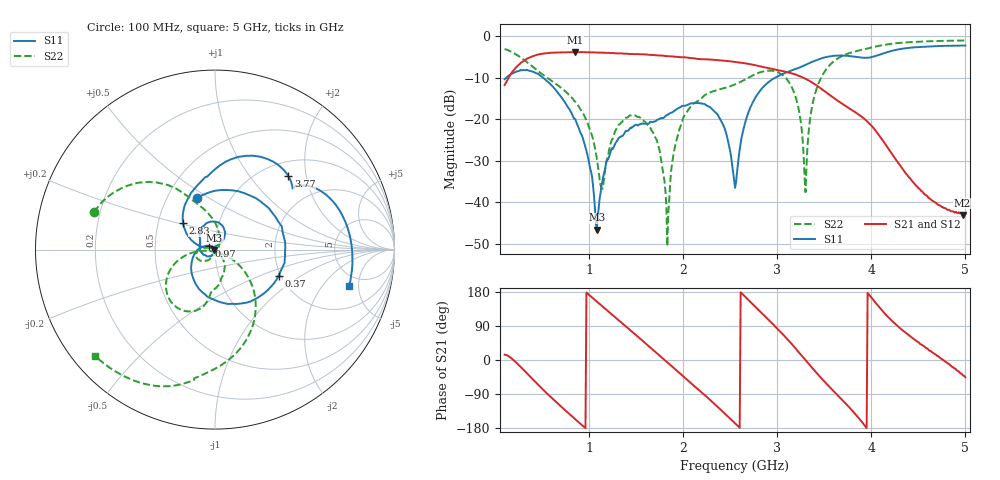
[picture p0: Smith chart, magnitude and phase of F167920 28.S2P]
!  2-Port S-parameters saved by WinCal
! VAR MeasName=S-Parameters (CALIBRATED_DATA) read from VNA (N5242A)
! VAR MeasDate=2016-11-22 9:56:32
! VAR NAME=F167920 28
! VAR FILENAME=F167920 28.S2P
! VAR DATE=2016-11-22 9:56:32
! VAR PHYS_PORTS=1,2
# Hz S DB R 50
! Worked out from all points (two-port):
!   491 points, 100 MHz to 5 GHz, reference 50 ohm
!   highest |S21| = -3.78 dB at 850 MHz (marker M1); lowest = -43.1 dB at 4.97 GHz (marker M2)
!   |S21| within 3 dB of the highest: 254.8 MHz to 2.725 GHz (2.47 GHz wide, 166 % of centre)
!   lowest |S11| = -46.7 dB at 1.08 GHz (marker M3), VSWR 1.01, Z = 49.6 - j0.172 ohm
!   |S11| at or under -10 dB: start of sweep to 116.4 MHz; 509.2 MHz to 2.976 GHz (2.466 GHz wide, 142 % of centre)
!   |S22| runs from -50.6 to -1.0 dB; largest |S21 - S12| = 0.0011
!   S11 on the Smith chart (normalised r, x): 100 MHz: 0.70, +0.45; 370 MHz: 1.95, -0.66; 970 MHz: 0.93, +0.04; 2.83 GHz: 0.67, +0.21; 3.77 GHz: 1.28, +1.58; 5 GHz: 3.77, -3.87
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1e8  -10.32 109.2  -11.75 14.3  -11.75 14.3  -3.05 162.8
3.7e8  -8.34 -22.4  -5.06 -43.5  -5.06 -43.4  -6.79 127.5
5.9e8  -11.57 -99.8  -3.96 -97.8  -3.95 -97.8  -10.61 113.7
8.5e8  -19.93 -177.9  -3.78 -156.1  -3.78 -156.1  -15.73 93.5
9.2e8  -23.80 164.6  -3.79 -171.1  -3.79 -171.1  -18.15 84.9
9.7e8  -27.62 149.8  -3.83 178.0  -3.83 178.0  -20.25 77.1
1.08e9  -46.65 -158.1  -3.90 154.4  -3.90 154.4  -29.36 45.7
1.14e9  -35.01 -107.6  -3.93 141.5  -3.93 141.5  -36.80 -39.0
1.3e9  -25.05 -137.6  -4.11 107.5  -4.11 107.5  -21.83 -129.5
1.74e9  -20.03 146.6  -4.60 13.4  -4.60 13.4  -26.86 165.8
1.83e9  -18.87 138.9  -4.77 -5.9  -4.76 -5.9  -50.63 -132.6
2.02e9  -16.75 115.5  -5.06 -47.4  -5.07 -47.4  -18.86 -62.1
2.37e9  -19.08 59.4  -5.74 -124.6  -5.75 -124.7  -12.87 -92.8
2.55e9  -36.55 102.8  -6.14 -166.9  -6.15 -166.9  -11.61 -96.9
2.83e9  -12.73 140.4  -7.28 124.8  -7.29 124.8  -8.58 -112.2
3.16e9  -8.16 100.8  -8.97 40.5  -8.98 40.5  -12.55 -161.0
3.3e9  -6.88 89.2  -10.23 -0.4  -10.24 -0.4  -37.60 -83.7
3.37e9  -6.14 83.2  -11.12 -20.6  -11.14 -20.6  -16.87 -31.8
3.77e9  -4.75 45.1  -17.44 -126.2  -17.47 -126.1  -4.01 -84.7
4.19e9  -3.66 31.4  -27.40 110.5  -27.44 110.8  -1.86 -109.3
4.97e9  -2.23 -14.0  -43.13 -39.3  -42.87 -37.8  -1.00 -137.6
5e9  -2.22 -15.4  -42.85 -45.8  -43.20 -44.3  -0.99 -138.3
